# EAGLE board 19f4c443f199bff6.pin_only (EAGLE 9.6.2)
REV: C

Size 35.56 x 17.78 mm. Coordinates in mm from the lower left corner, seen from the top.
Outline: 0,6.35 0,1.27 arc90 1.27,0 34.29,0 arc90 35.56,1.27 35.56,16.51 arc90 34.29,17.78 1.27,17.78 arc90 0,16.51 0,11.68 0.51,11.18 0.51,6.86 0,6.35
Copper layers (1*16): Top 0.035mm / dielectric 1.5mm / Bottom 0.035mm
Design rules "adafruit 7-7 *": minimum track width 6mil, minimum drill 15.5mil, track to track 8mil, track to pad 7mil, pad to pad 7mil, via to via 7mil, smd to smd 7mil, copper to edge 10mil, drill to drill 8mil, minimum pad ring 10mil, minimum via ring 8mil, stop-mask expansion 2mil, vias tented up to drill 20mil, thermal gap 10mil
Net classes: 1 power: width 0.305 mm

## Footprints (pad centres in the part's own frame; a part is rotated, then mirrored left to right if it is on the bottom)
_0603MP = smd 0.8 x 0.8: 1 -0.762,0; 2 0.762,0
_0402NO = smd 0.6 x 0.6: 1 -0.508,0; 2 0.508,0
0805-NO = smd 1.24 x 1.5: 1 -0.95,0; 2 0.95,0
SOD-323F = smd 1 x 0.8: A -1,0; C 1,0
SC70-5 = smd 0.4 x 0.7: 1 -0.65,-0.85; 2 0,-0.85; 3 0.65,-0.85; 4 0.65,0.85; 5 -0.65,0.85
QFN56_7MM_REDUCEDEPAD = smd 0.875 x 0.2: 1 -3.45,2.6; 2 -3.45,2.2; 3 -3.45,1.8; 4 -3.45,1.4; 5 -3.45,1; 6 -3.45,0.6; 7 -3.45,0.2; 8 -3.45,-0.2; 9 -3.45,-0.6; 10 -3.45,-1; 11 -3.45,-1.4; 12 -3.45,-1.8; 13 -3.45,-2.2; 14 -3.45,-2.6; 29 3.45,-2.6; 30 3.45,-2.2; 31 3.45,-1.8; 32 3.45,-1.4; 33 3.45,-1; 34 3.45,-0.6; 35 3.45,-0.2; 36 3.45,0.2; 37 3.45,0.6; 38 3.45,1; 39 3.45,1.4; 40 3.45,1.8; 41 3.45,2.2; 42 3.45,2.6 | smd 0.2 x 0.875: 15 -2.6,-3.45; 16 -2.2,-3.45; 17 -1.8,-3.45; 18 -1.4,-3.45; 19 -1,-3.45; 20 -0.6,-3.45; 21 -0.2,-3.45; 22 0.2,-3.45; 23 0.6,-3.45; 24 1,-3.45; 25 1.4,-3.45; 26 1.8,-3.45; 27 2.2,-3.45; 28 2.6,-3.45; 43 2.6,3.45; 44 2.2,3.45; 45 1.8,3.45; 46 1.4,3.45; 47 1,3.45; 48 0.6,3.45; 49 0.2,3.45; 50 -0.2,3.45; 51 -0.6,3.45; 52 -1,3.45; 53 -1.4,3.45; 54 -1.8,3.45; 55 -2.2,3.45; 56 -2.6,3.45 | smd 3.2 x 3.2: P$1 0,0
1X05_ROUND_70 = drill 1 pad 1.778: 1 -5.08,0; 2 -2.54,0; 3 0,0; 4 2.54,0; 5 5.08,0
1X14_ROUND70 = drill 1 pad 1.676: 1 -16.51,0; 2 -13.97,0; 3 -11.43,0; 4 -8.89,0; 5 -6.35,0; 6 -3.81,0; 7 -1.27,0; 8 1.27,0; 9 3.81,0; 10 6.35,0; 11 8.89,0; 12 11.43,0; 13 13.97,0; 14 16.51,0
CHIPLED_0603_NOOUTLINE = smd 0.8 x 0.8: A 0,-0.75; C 0,0.75
SK6805_1515 = smd 0.5 x 0.5: 1 -0.5,-0.45; 2 0.5,-0.45; 3 0.5,0.45; 4 -0.5,0.45
BTN_KMR2_4.6X2.8 = smd 0.9 x 0.9: A 2.05,0.8; A' -2.05,0.8; B 2.05,-0.8; B' -2.05,-0.8
TESTPOINT_ROUND_1.5MM_NO = smd 1.5 x 1.5: P$1 0,0
USON8_4X4 = smd 0.6 x 0.4: 1 -1.85,1.2; 2 -1.85,0.4; 3 -1.85,-0.4; 4 -1.85,-1.2; 5 1.85,-1.2; 6 1.85,-0.4; 7 1.85,0.4; 8 1.85,1.2 | smd 2 x 3: PAD 0,0
SOT23-5 = smd 0.55 x 1.2: 1 -0.95,-1.3; 2 0,-1.3; 3 0.95,-1.3; 4 0.95,1.3; 5 -0.95,1.3
FIDUCIAL_1MM = smd 1 x 1: 1 0,0
4UCONN_20329_NARROW = smd 1 x 2: BASE@1 -0.75,-2; BASE@2 0.75,-2 | smd 0.4 x 1.35: D+ 0,0.775; D- -0.65,0.775; GND 1.3,0.775; ID 0.65,0.775; VBUS -1.3,0.775 | drill 0.8 pad 1.27 octagon: SPRT@1 -3.3,0.9; SPRT@2 3.3,0.9 | drill 0.9 pad 2.413 square: SPRT@3 -3.6,-1.9; SPRT@4 3.6,-1.9 | hole 0.7: -1.95,0; 1.95,0
CRYSTAL_2.5X2 = smd 0.9 x 0.75: 1 -0.825,-0.625; 2 0.825,-0.625; 3 0.825,0.625; 4 -0.825,0.625

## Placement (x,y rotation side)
C2  1uF  [_0603MP]  25.08,13.77 0 top
C3  0.1uF  [_0402NO]  24.68,5.38 90 top
C4  0.1uF  [_0402NO]  13.09,6.25 0 top
C6  10µF  [0805-NO]  8.51,12.03 90 top
C8  10µF  [0805-NO]  8.83,4.11 180 top
C10  0.1uF  [_0402NO]  26.73,6.22 180 top
C11  1uF  [_0603MP]  25.97,4.53 270 top
C12  0.1uF  [_0402NO]  11.24,4.51 90 top
C13  0.1uF  [_0402NO]  13.09,7.47 180 top
C16  0.1uF  [_0402NO]  24.51,3.8 0 top
C19  22pF  [_0402NO]  11.7,12.19 0 top
C20  22pF  [_0402NO]  11.42,8.14 90 top
D1  NSR0320  [SOD-323F]  5.61,13.89 0 top
D2  NSR0320  [SOD-323F]  6.99,11.8 90 top
D3  NSR0320  [SOD-323F]  32.33,9.45 90 top
IC1  74HCT1G125DBV  [SC70-5]  13.97,13.08 0 top
IC3  RP2040_QFN56  [QFN56_7MM_REDUCEDEPAD]  20.51,9.21 270 top
JP1  [1X05_ROUND_70]  34.29,8.89 90 top
JP2  [1X14_ROUND70]  17.78,16.51 0 top
JP4  [1X14_ROUND70]  17.78,1.27 180 top
L  RED  [CHIPLED_0603_NOOUTLINE]  9.88,12.02 180 top
LED1  WS2812B_SK6805_1515  [SK6805_1515]  13.09,4.9 90 top
R1  10K  [_0402NO]  8.6,9.78 180 top
R2  10k  [_0402NO]  25.3,12.64 0 top
R3  22  [_0402NO]  6.73,6.29 270 top
R4  22  [_0402NO]  6.83,9.22 270 top
R5  10K  [_0402NO]  5.91,3.94 180 top
R6  1K  [_0402NO]  13.04,8.62 0 top
R7  1K  [_0402NO]  11.24,13.8 180 top
R11  1K  [_0402NO]  31.79,7.29 0 top
SW2  KMR2  [BTN_KMR2_4.6X2.8]  30.23,4.95 180 top
SW3  KMR2  [BTN_KMR2_4.6X2.8]  30.23,12.83 180 top
TP1  [TESTPOINT_ROUND_1.5MM_NO]  29.21,11.43 0 bottom
U1  GD25x16  [USON8_4X4]  28.46,8.76 180 top
U2  AP2112K-3.3  [SOT23-5]  9.02,7.24 180 top
U$4  [ITSY2040_TOP]  0,0 0 top
U$5  [ITSY2040_BOT]  35.56,0 0 bottom
U$34  FIDUCIAL_1MM  [FIDUCIAL_1MM]  30.61,12.95 270 top
U$35  FIDUCIAL_1MM  [FIDUCIAL_1MM]  0.81,3.17 270 top
X3  microUSB  [4UCONN_20329_NARROW]  4.45,8.89 270 top
Y1  12MHZ  [CRYSTAL_2.5X2]  12,10.46 0 top

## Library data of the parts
C2-C4 C6 C10-C13 C16 C19 C20 JP1 JP2 JP4 L LED1 R1-R7 R11 SW2 SW3 TP1 U1 U2 Y1 = microbuilder
C8 = microbuilder; COMPANY: ADAFRUIT INDUSTRIES; DRAWN: KTOWN; REV: A
D1-D3 = adafruit
IC1 = 74xx-little-us
IC3 = adafruit_micro
U$4 U$5 = itsy_silks
U$34 U$35 = microbuilder; BOM: EXCLUDE
X3 = adafruit_connector

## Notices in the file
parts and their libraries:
microbuilder: This work is placed in the public domain, and may be freely used for commercial and non-commercial work with the following conditions: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
